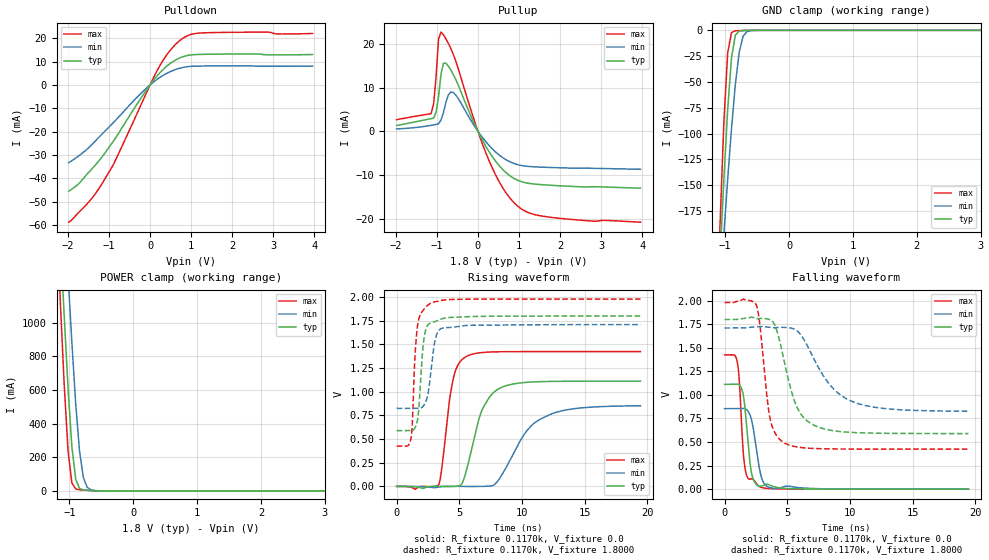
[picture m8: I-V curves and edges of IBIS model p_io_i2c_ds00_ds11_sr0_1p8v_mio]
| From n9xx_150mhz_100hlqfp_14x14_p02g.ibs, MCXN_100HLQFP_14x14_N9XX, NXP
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[Model] p_io_i2c_ds00_ds11_sr0_1p8v_mio
|   Model p_io_i2c_ds00_ds11_sr0_1p8v_mio
| This model was characterised for following simulation conditions:
| External (pad) voltage:
|   - Typ: 1.8V,   - Min: 1.71V,   - Max: 1.98V
| Library cells for typ/min/max conditions are connected as defined below:
|  pad - External Pad
|  ipp_do_lv - Core Input
|  ipp_obe_lv - Output Buffer Enable
|  IOGC - NC
|  REFH3V3 - REFH3V3
|  REFL3V3 - REFL3V3
|  ZI - NC
|  abut_ncal_vddio[1] - vssio vddio vddio
|  abut_ncal_vddio[2] - vddio vddio vssio
|  abut_ncal_vddio[3] - vddio
|  abut_ncal_vddio[4] - vssio vddio vddio
|  abut_ncal_vddio[5] - vddio vddio vssio
|  abut_ncal_vddio[6] - vddio
|  abut_pcal_vddio[1] - vssio
|  abut_pcal_vddio[2] - vddio vssio vddio
|  abut_pcal_vddio[3] - vssio
|  abut_pcal_vddio[4] - vssio
|  abut_pcal_vddio[5] - vddio vssio vddio
|  abut_pcal_vddio[6] - vssio
|  ipp_do_1p8v - ipp_do_1p8v
|  ipp_dse_lv[0] - 0
|  ipp_dse_lv[1] - vdd_lv
|  ipp_eftd_lv - NC
|  ipp_ina_mux_vddio - NC
|  ipp_ina_mux_vddio[0] - NC
|  ipp_ina_mux_vddio[1] - NC
|  ipp_ina_r0_vddio - NC
|  ipp_ina_r0a_vddio - NC
|  ipp_ina_r0b_vddio - NC
|  ipp_ina_r0c_vddio - NC
|  ipp_ina_r0d_vddio - NC
|  ipp_ina_r0e_vddio - NC
|  ipp_ina_r0f_vddio - NC
|  ipp_ina_r300_vddio - NC
|  ipp_ina_r300a_vddio - NC
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Model_type I/O
Polarity   Non-Inverting
Enable   Active-High
Vinl =   0.5400V
Vinh =   1.2600V
Vmeas =  0.9000V
Cref =   30.0000pF
Rref =   1.0000M
Vref =   1.8000V
C_comp   1.4328pF   1.3910pF   1.4871pF
|C_comp_pullup   0.6294pF   0.6727pF   0.5892pF
|C_comp_pulldown   0.7022pF   0.7084pF   0.7046pF
[Model Spec]
| variable   typ   min   max
Vinh   1.2600V   1.1970V   1.3860V
Vinl   0.5400V   0.5130V   0.5940V
[Temperature Range]   25.0000   0.1250k   -40.0000
[Voltage Range]   1.8000V   1.7100V   1.9800V
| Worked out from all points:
|   slope of the pulldown table from 0 to 0.27 V, typ, clamps not added: 46.9 ohm
|   slope of the pullup table from 0 to 0.27 V, typ, clamps not added: 58.1 ohm
|   GND clamp passes 1 mA (typ) near -0.78 V on its own axis
|   POWER clamp passes 1 mA (typ) near -0.58 V on its own axis
|   rising waveform, R_fixture 0.1170k, V_fixture 0.0: 20-80 % time 1.48ns typ, 2.5ns min, 826ps max; typ from 0 V to 1.11 V
|   rising waveform, R_fixture 0.1170k, V_fixture 1.8000: 20-80 % time 403ps typ, 513ps min, 362ps max; typ from 0.59 V to 1.8 V
|   falling waveform, R_fixture 0.1170k, V_fixture 0.0: 20-80 % time 478ps typ, 617ps min, 385ps max; typ from 1.11 V to 0 V
|   falling waveform, R_fixture 0.1170k, V_fixture 1.8000: 20-80 % time 1.5ns typ, 2.65ns min, 777ps max; typ from 1.8 V to 0.59 V
[Pulldown]
|Voltage   I(typ)   I(min)   I(max)
-1.98V    -45.46mA   -33.22mA   -58.69mA
-1.74V    -42.29mA   -30.37mA   -54.55mA
-1.5V     -37.49mA   -26.94mA   -50.24mA
-1.14V    -30.1mA    -20.51mA   -41.41mA
-840mV    -22.72mA   -15.13mA   -32.11mA
-240mV    -6.149mA   -3.914mA   -9.292mA
180mV     4.04mA     2.499mA    6.393mA
420mV     8.21mA     5.083mA    13.17mA
720mV     11.54mA    7.145mA    18.92mA
960mV     12.77mA    7.907mA    21.41mA
1.26V     13.1mA     8.11mA     22.25mA
3.96V     13.03mA    8.089mA    22.03mA
[Pullup]
|Voltage   I(typ)   I(min)   I(max)
-1.98V    1.322mA    535.1uA    2.661mA
-1.14V    2.892mA    1.357mA    4.033mA
-1.08V    2.998mA    1.458mA    6.209mA
-1.02V    4.373mA    1.562mA    12.42mA
-960mV    7.844mA    1.723mA    21.06mA
-900mV    13.06mA    2.576mA    22.72mA
-780mV    15.6mA     6.622mA    21.17mA
-600mV    13mA       8.883mA    17.6mA
240mV     -4.193mA   -2.919mA   -6.042mA
900mV     -10.91mA   -7.454mA   -16.56mA
1.62V     -12.28mA   -8.246mA   -19.51mA
3.96V     -13.04mA   -8.71mA    -20.83mA
[GND_clamp]
|Voltage   I(typ)   I(min)   I(max)
-1.98V    -1.586A    -1.229A    -2.1A
-1.08V    -221.4mA   -253.6mA   -188.5mA
-1.02V    -144.6mA   -197.7mA   -89.32mA
-960mV    -76.59mA   -144.3mA   -21.58mA
-900mV    -26.43mA   -94.89mA   -2.183mA
-840mV    -4.754mA   -52.29mA   -428.7uA
-780mV    -708.9uA   -21.31mA   -240uA
-720mV    -194.5uA   -5.864mA   -159.9uA
-660mV    -97.62uA   -1.274mA   -100.6uA
-600mV    -55.49uA   -286.4uA   -56.47uA
-420mV    -4.265uA   -10.7uA    -2.74uA
3.96V     0A         0A         0A
[POWER_clamp]
|Voltage   I(typ)   I(min)   I(max)
-1.98V    7.929A     7.752A     8.366A
-1.2V     1.949A     2.483A     1.628A
-1.14V    1.495A     2.081A     1.12A
-1.08V    1.044A     1.68A      633.7mA
-1.02V    613.2mA    1.282A     240.4mA
-960mV    264mA      886.2mA    47.43mA
-900mV    69.94mA    519.6mA    11.58mA
-840mV    15.1mA     237.3mA    7.049mA
-780mV    5.589mA    78.54mA    5.099mA
-720mV    3.316mA    21.56mA    3.521mA
-660mV    2.102mA    6.487mA    2.205mA
3.96V     0A         0A         0A
[Ramp]
| variable   typ   min   max
dV/dt_r  0.6673/1.4769n   0.5112/2.4989n   0.8549/0.8260n
dV/dt_f  0.7261/1.4957n   0.5300/2.6523n   0.9330/0.7775n
R_load = 0.1170k
[Rising Waveform]
R_fixture= 0.1170k
V_fixture= 0.0
V_fixture_min= 0.0
V_fixture_max= 0.0
|time   V(typ)   V(min)   V(max)
0s        403.1pV    155.9nV    14.26pV
3.357ns   480.9uV    -6.73mV    19.92mV
4.492ns   -1.247mV   1.033mV    1.126V
5.152ns   18.55mV    215.6uV    1.331V
5.56ns    165.9mV    -981.8uV   1.373V
6.783ns   797.8mV    -593.2uV   1.414V
8.201ns   1.036V     81.36mV    1.423V
10.21ns   1.098V     557mV      1.425V
11.52ns   1.107V     714.7mV    1.425V
19.45ns   1.112V     852.1mV    1.425V
[Rising Waveform]
R_fixture= 0.1170k
V_fixture= 1.8000
V_fixture_min= 1.7100
V_fixture_max= 1.9800
|time   V(typ)   V(min)   V(max)
0s        589.7mV    824.4mV    425mV
1.141ns   589.4mV    824.4mV    505.4mV
1.25ns    591.3mV    824.4mV    656.7mV
1.582ns   658mV      824.2mV    1.597V
1.751ns   793.6mV    824.3mV    1.76V
2.169ns   1.551V     856.2mV    1.871V
2.639ns   1.724V     1.107V     1.93V
3.067ns   1.742V     1.547V     1.952V
3.636ns   1.772V     1.673V     1.968V
19.45ns   1.8V       1.71V      1.98V
[Falling Waveform]
R_fixture= 0.1170k
V_fixture= 0.0
V_fixture_min= 0.0
V_fixture_max= 0.0
|time   V(typ)   V(min)   V(max)
0s        1.112V     854.4mV    1.425V
996.5ps   1.114V     854.3mV    1.36V
1.17ns    1.107V     854.7mV    1.166V
1.373ns   1.062V     856.2mV    653.5mV
1.529ns   970.5mV    856.3mV    333.1mV
1.743ns   694.5mV    845.7mV    152.7mV
2.162ns   165mV      730.8mV    111.7mV
2.81ns    32.85mV    198.8mV    25.27mV
3.952ns   25.88mV    7.847mV    4.068mV
19.45ns   2.55uV     27.88uV    207.5nV
[Falling Waveform]
R_fixture= 0.1170k
V_fixture= 1.8000
V_fixture_min= 1.7100
V_fixture_max= 1.9800
|time   V(typ)   V(min)   V(max)
0s        1.8V       1.71V      1.98V
2.54ns    1.811V     1.723V     1.952V
2.8ns     1.81V      1.726V     1.761V
3.63ns    1.797V     1.716V     750.8mV
4.112ns   1.707V     1.713V     576.4mV
4.744ns   1.365V     1.717V     493.2mV
5.81ns    859.7mV    1.677V     447mV
7.381ns   663.5mV    1.316V     430.2mV
10.81ns   598mV      901.5mV    425.4mV
19.45ns   589.9mV    826.7mV    425mV
